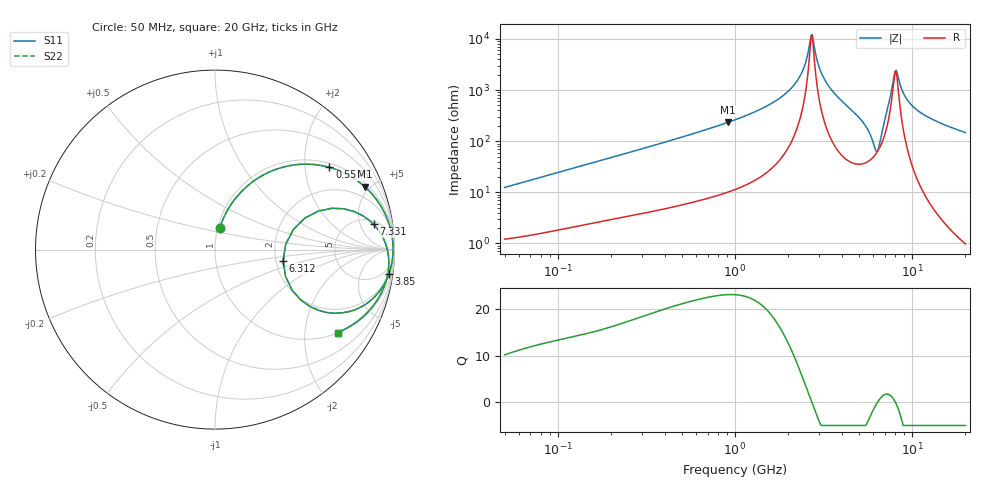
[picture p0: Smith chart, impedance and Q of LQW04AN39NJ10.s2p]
!Murata Part Number: LQW04AN39NJ10
!These Parameters are Measured in Series Mode Connection
!  o--[Z]--o
!Port1  Port2
!  o-------o
!Freq. Start=50[MHz] Stop=20[GHz], 401[Steps]
# Hz S RI R 50
!Freq.(Hz) S11(Real) S11(Imag) S21(Real) S21(Imag) S12(Real) S12(Imag) S22(Real) S22(Imag)
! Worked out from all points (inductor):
!   401 points, 50 MHz to 20 GHz, reference 50 ohm
!   read as one part in series: L = 39.2 nH near 51.52 MHz
!   highest Q = 23.2 at 914 MHz (marker M1), where L = 40.7 nH
!   self-resonance near 2.687 GHz
!   S11 on the Smith chart (normalised r, x): 50 MHz: 1.02, +0.25; 557.6 MHz: 1.12, +2.68; 3.85 GHz: 2, -14; 6.312 GHz: 2.19, -0.33; 7.331 GHz: 6, +8; 20 GHz: 1.02, -2.94
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5e7  0.0265 0.119  0.9735 -0.119  0.9735 -0.119  0.0265 0.119
1.364002e8  0.114 0.2853  0.886 -0.2853  0.886 -0.2853  0.114 0.2853
3.721004e8  0.442 0.4719  0.558 -0.4719  0.558 -0.4719  0.442 0.4719
5.575697e8  0.637 0.4584  0.363 -0.4584  0.363 -0.4584  0.637 0.4584
9.140482e8  0.8351 0.3501  0.1649 -0.3501  0.1649 -0.3501  0.8351 0.3501
1e9  0.8622 0.3237  0.1378 -0.3237  0.1378 -0.3237  0.8622 0.3237
2.05233e9  0.983 0.0936  0.017 -0.0936  0.017 -0.0936  0.983 0.0936
2.383959e9  0.9903 0.0441  0.00972 -0.0441  0.00972 -0.0441  0.9903 0.0441
2.728004e9  0.9921 -0.00188  0.0079 0.00188  0.0079 0.00188  0.9921 -0.00188
3.121702e9  0.9888 -0.0503  0.0112 0.0503  0.0112 0.0503  0.9888 -0.0503
3.850025e9  0.9686 -0.1357  0.0314 0.1357  0.0314 0.1357  0.9686 -0.1357
4.966507e9  0.874 -0.2778  0.126 0.2778  0.126 0.2778  0.874 -0.2778
5.683258e9  0.6713 -0.3546  0.3287 0.3546  0.3287 0.3546  0.6713 -0.3546
6.311513e9  0.3794 -0.0635  0.6206 0.0635  0.6206 0.0635  0.3794 -0.0635
6.802353e9  0.6497 0.2301  0.3503 -0.2301  0.3503 -0.2301  0.6497 0.2301
7.331367e9  0.8833 0.1411  0.1167 -0.1411  0.1167 -0.1411  0.8833 0.1411
7.442007e9  0.9055 0.1153  0.0945 -0.1153  0.0945 -0.1153  0.9055 0.1153
7.901521e9  0.9535 0.0235  0.0465 -0.0235  0.0465 -0.0235  0.9535 0.0235
8.141811e9  0.9631 -0.0145  0.0369 0.0145  0.0369 0.0145  0.9631 -0.0145
9.178299e9  0.9641 -0.1288  0.0359 0.1288  0.0359 0.1288  0.9641 -0.1288
1.050288e10  0.9379 -0.2181  0.0621 0.2181  0.0621 0.2181  0.9379 -0.2181
2e10  0.6829 -0.462  0.3171 0.462  0.3171 0.462  0.6829 -0.462
